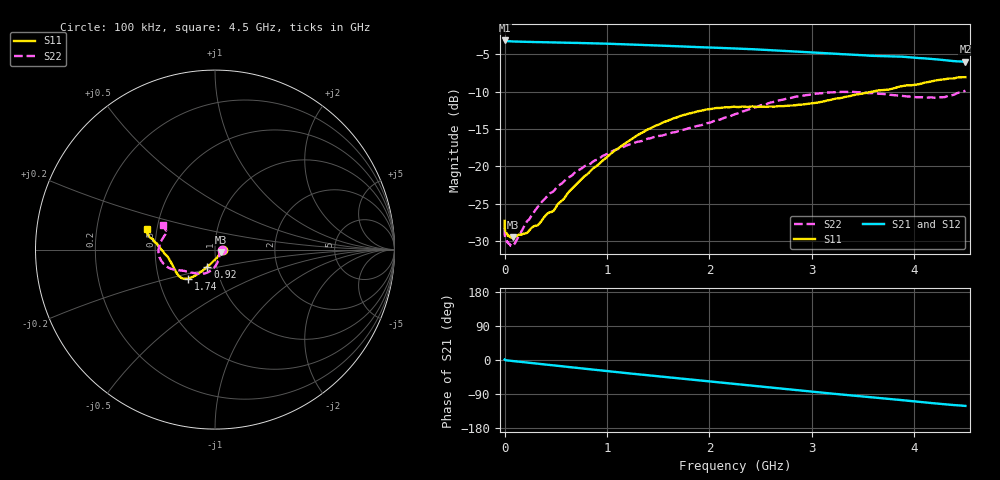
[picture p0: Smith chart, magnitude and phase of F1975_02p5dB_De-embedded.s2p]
! Integrated Device Technology
! Corporate Headquarters
! 6024 Silver Creek Valley Road
! San Jose, CA 95138  USA
! Phone:  1-408-284-8200
! Toll Free:  1-800-223-1366
! Webpage:  http://www.idt.com/
! Timing and RF Division
! 515 Groton Road, Suite 102
! Westford, MA 01886-6024
! Device:  F1975
! Description: 6-bit, 75 ohm, 0.5 dB Digital Step Attenuator
! Frequency:  5.0 MHz -  3.00 GHz
! Package:  4x4 mm QFN Plastic Package: 20 pin
! Ports:  2 RF, 11 DC
!  Pin  1  = D5 (16 dB)
!  Pin  2  = RF1  =  Port 1
!  Pin  3  = Serial Data In (DATA)
!  Pin  4  = Serial Clock (CLK)
!  Pin  5  = Serial Latch Enable (LE)
!  Pin  6  = VDD
!  Pin  7  = NC
!  Pin  8  = NC
!  Pin  9  = NC
!  Pin 10  = GND
!  Pin 11  = GND
!  Pin 12  = NC
!  Pin 13  = VMODE
!  Pin 14  = RF2  =  Port 2
!  Pin 15  = D4 (8 dB)
!  Pin 16  = D3 (4 dB)
!  Pin 17  = D2 (2 dB)
!  Pin 18  = NC
!  Pin 19  = D1 (1 dB)
!  Pin 20  = D0 (0.5 dB)
! State:  5
! Atten State:  2.5 dB
! Voltage:  +3.30 Volts
! Current:  0.564 mA
! Data:  The device was measured on a F1975 evaluation board which has
!  individual transmission lines to the RF pins.  Data was collected
!  using a calibrated network analyzer.  The evaluation board was
!  de-embedded using Automatic Fixture Removal (AFR).
!  The reference plane is the edge of the package pin.
! Misc:
!  Action Tracker AT0415
! Date Measured:  2018-02-08
! Date:  2018-03-26  MJV
! Note:
!  Integrated Device Technology supplies this data as a sample of measured
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# GHz S dB R 75
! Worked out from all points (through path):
!   291 points, 100 kHz to 4.5 GHz, reference 75 ohm
!   highest |S21| = -3.15 dB at 100 kHz (marker M1); lowest = -6.0 dB at 4.5 GHz (marker M2)
!   group delay of S21, straight-line fit = 75.8 ps
!   lowest |S11| = -29.5 dB at 80 MHz (marker M3), VSWR 1.07, Z = 79.7 - j2.07 ohm
!   |S11| at or under -10 dB: start of sweep to 3.595 GHz
!   |S22| runs from -30.7 to -9.9 dB; largest |S21 - S12| = 0.00025
!   S11 on the Smith chart (normalised r, x): 100 kHz: 1.09, +0.00; 920 MHz: 0.90, -0.17; 1.74 GHz: 0.71, -0.24; 4.5 GHz: 0.44, +0.12
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0.0001  -27.33 0.0  -3.15 1.2  -3.15 1.2  -28.31 0.6
0.0005  -27.89 -2.1  -3.18 1.1  -3.17 1.1  -28.70 -1.0
0.002  -28.33 -2.1  -3.20 0.8  -3.20 0.8  -29.23 -1.5
0.019  -28.95 -7.7  -3.24 -0.8  -3.24 -0.8  -30.05 -9.6
0.08  -29.55 -22.9  -3.28 -2.7  -3.28 -2.7  -30.71 -27.7
0.22  -28.93 -48.8  -3.34 -6.8  -3.34 -6.8  -27.35 -55.4
0.36  -27.33 -71.1  -3.38 -10.8  -3.38 -10.9  -24.84 -68.3
0.42  -26.33 -77.2  -3.40 -12.6  -3.40 -12.6  -23.94 -72.3
0.48  -25.94 -84.8  -3.41 -14.3  -3.41 -14.3  -23.33 -76.6
0.62  -23.56 -99.1  -3.46 -18.3  -3.46 -18.3  -21.51 -84.3
0.76  -21.61 -107.0  -3.50 -22.3  -3.50 -22.3  -20.22 -91.3
0.92  -19.73 -114.1  -3.55 -26.9  -3.55 -26.9  -18.98 -98.9
1.28  -16.00 -124.2  -3.71 -37.1  -3.71 -37.1  -16.81 -113.4
1.52  -14.32 -128.6  -3.83 -43.8  -3.83 -43.8  -15.92 -122.5
1.74  -13.17 -132.6  -3.96 -49.8  -3.96 -49.8  -15.14 -131.4
2.26  -12.05 -145.3  -4.23 -63.8  -4.23 -63.8  -12.99 -148.6
2.68  -11.94 -159.4  -4.50 -75.2  -4.50 -75.2  -11.18 -158.2
3.02  -11.55 -170.4  -4.76 -84.1  -4.76 -84.1  -10.34 -167.6
3.4  -10.49 -180.0  -5.06 -93.7  -5.06 -93.7  -10.03 180.0
3.76  -9.70 173.9  -5.28 -102.6  -5.28 -102.5  -10.43 169.8
4.22  -8.48 168.5  -5.67 -115.0  -5.67 -115.0  -10.83 159.1
4.5  -8.07 163.3  -5.98 -121.2  -5.98 -121.2  -9.87 155.3
